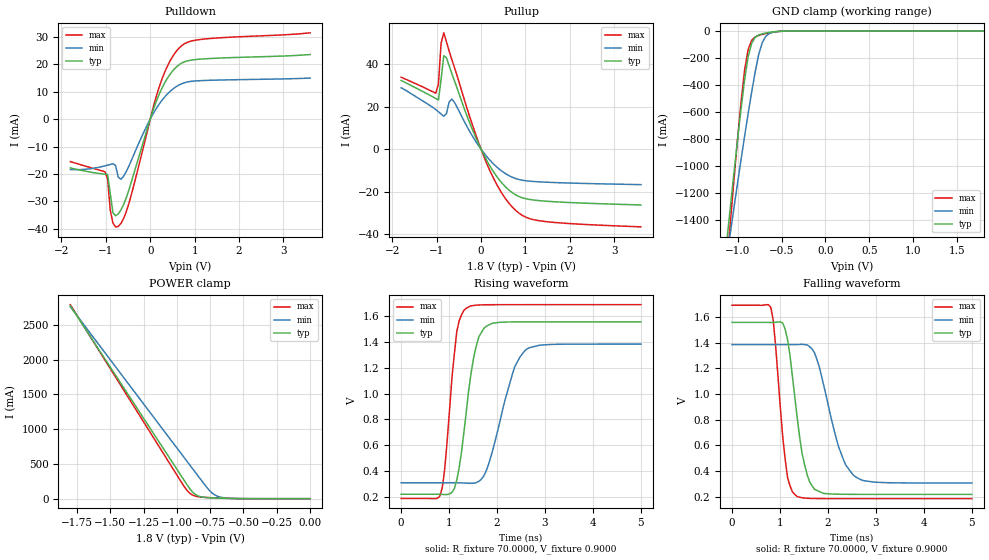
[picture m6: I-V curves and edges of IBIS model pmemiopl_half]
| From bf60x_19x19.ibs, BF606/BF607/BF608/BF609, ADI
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[Model]  pmemiopl_half
Model_type I/O
Polarity   Non-Inverting
Enable   Active-Low
Vinl =   0.6500V
Vinh =   1.1500V
Vmeas =  0.9000V
Cref =   5.0000pF
Rref =   70.0000
Vref =   0.9000V
C_comp   3.6123pF   3.9509pF   3.3683pF
[Temperature Range]   25.0000   0.1250k   0.0
[Voltage Range]   1.8000V   1.7000V   1.9000V
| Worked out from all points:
|   slope of the pulldown table from 0 to 0.27 V, typ, clamps not added: 23.5 ohm
|   slope of the pullup table from 0 to 0.27 V, typ, clamps not added: 26.3 ohm
|   GND clamp passes 1 mA (typ) near -0.49 V on its own axis
|   POWER clamp passes 1 mA (typ) near -0.53 V on its own axis
|   rising waveform, R_fixture 70.0000, V_fixture 0.9000: 20-80 % time 283ps typ, 455ps min, 208ps max; typ from 0.219 V to 1.56 V
|   falling waveform, R_fixture 70.0000, V_fixture 0.9000: 20-80 % time 280ps typ, 443ps min, 205ps max; typ from 1.56 V to 0.219 V
[Pulldown]
|Voltage   I(typ)   I(min)   I(max)
-1.8V     -17.81mA   -18.4mA    -15.51mA
-1.02V    -20.1mA    -17.05mA   -19.21mA
-960mV    -20.2mA    -16.81mA   -21.87mA
-900mV    -27.22mA   -16.55mA   -33.33mA
-840mV    -34.17mA   -16.26mA   -37.96mA
-780mV    -35.26mA   -16.94mA   -39.32mA
-720mV    -34.59mA   -21.21mA   -39.17mA
-480mV    -25.82mA   -17.09mA   -30.75mA
240mV     10.49mA    6.362mA    13.53mA
660mV     19.97mA    12.55mA    26.11mA
1.2V      21.98mA    14.09mA    29.19mA
3.6V      23.58mA    14.99mA    31.5mA
[Pullup]
|Voltage   I(typ)   I(min)   I(max)
-1.8V     32.34mA    28.88mA    33.85mA
-1.02V    23.85mA    18.64mA    26.32mA
-960mV    23.13mA    17.63mA    30.81mA
-900mV    32.98mA    16.53mA    49.91mA
-840mV    44.01mA    15.49mA    54.74mA
-660mV    35.66mA    23.59mA    42.27mA
-240mV    11.52mA    7.772mA    14.28mA
120mV     -4.955mA   -3.244mA   -6.328mA
420mV     -14.66mA   -9.536mA   -19.06mA
720mV     -20.68mA   -13.33mA   -27.57mA
1.32V     -24.2mA    -15.36mA   -33.65mA
3.6V      -26.22mA   -16.66mA   -36.51mA
[GND_clamp]
|Voltage   I(typ)   I(min)   I(max)
-1.8V     -6.07A     -4.897A    -7.407A
-1.12V    -1.546A    -1.671A    -1.719A
-1.08V    -1.294A    -1.488A    -1.405A
-1V       -805.6mA   -1.129A    -801.4mA
-960mV    -575.4mA   -952.7mA   -523.3mA
-920mV    -361.5mA   -780.6mA   -288.5mA
-880mV    -190.9mA   -613.7mA   -138.4mA
-840mV    -90.93mA   -454mA     -68.72mA
-800mV    -46.73mA   -305.2mA   -43.97mA
-720mV    -20.7mA    -86.99mA   -25.13mA
-600mV    -6.426mA   -9.601mA   -8.755mA
1.8V      90.38pA    38.35nA    69.58pA
[POWER_clamp]
|Voltage   I(typ)   I(min)   I(max)
-1.8V     2.775A     2.761A     2.791A
-960mV    306.4mA    628.6mA    218.5mA
-920mV    189.6mA    527.3mA    109.9mA
-900mV    135.2mA    476.7mA    73.19mA
-880mV    91.17mA    426mA      49.38mA
-840mV    39.16mA    324.6mA    27.86mA
-760mV    13.35mA    127mA      16mA
-720mV    9.728mA    59.79mA    12.42mA
-680mV    7.06mA     25.51mA    9.286mA
-540mV    1.159mA    1.976mA    1.7mA
0V        90.38pA    3.773nA    81.3pA
[Ramp]
| variable   typ   min   max
dV/dt_r  0.6316/0.3291n   0.4413/0.4867n   0.7626/0.2367n
dV/dt_f  0.6255/0.3881n   0.4177/0.5365n   0.7652/0.2903n
R_load = 50.0000
[Rising Waveform]
R_fixture= 70.0000
V_fixture= 0.9000
V_fixture_min= 0.8500
V_fixture_max= 0.9500
L_fixture= 0.0H
C_fixture= 0.0F
|time   V(typ)   V(min)   V(max)
0s        218.8mV    307.4mV    185.5mV
810ps     218.3mV    307.4mV    205.3mV
910ps     216.1mV    307.4mV    420mV
1.16ns    328.6mV    307.3mV    1.48V
1.36ns    863.1mV    304.6mV    1.663V
1.52ns    1.296V     304.3mV    1.684V
1.72ns    1.504V     358.2mV    1.69V
2.37ns    1.556V     1.209V     1.69V
2.63ns    1.557V     1.348V     1.691V
5ns       1.557V     1.384V     1.691V
[Falling Waveform]
R_fixture= 70.0000
V_fixture= 0.9000
V_fixture_min= 0.8500
V_fixture_max= 0.9500
L_fixture= 0.0H
C_fixture= 0.0F
|time   V(typ)   V(min)   V(max)
0s        1.557V     1.385V     1.691V
810ps     1.556V     1.384V     1.674V
1.06ns    1.552V     1.385V     659.5mV
1.16ns    1.421V     1.384V     348.6mV
1.36ns    815.1mV    1.385V     202.2mV
1.52ns    441.1mV    1.384V     190mV
1.72ns    258.7mV    1.322V     186.9mV
2.22ns    220.4mV    592.5mV    185.6mV
2.58ns    219.1mV    354.3mV    185.5mV
5ns       218.8mV    307.4mV    185.5mV
